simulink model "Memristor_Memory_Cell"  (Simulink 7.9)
settings: Solver=ode113  StartTime=0.0  StopTime=10.0  RelTol=3e-14
undefined symbols (not defined in the file or in its folder): sigbuilder_block
libraries: fl_lib x11, nesl_utility x5, Memristor_lib x1, elec_lib x1

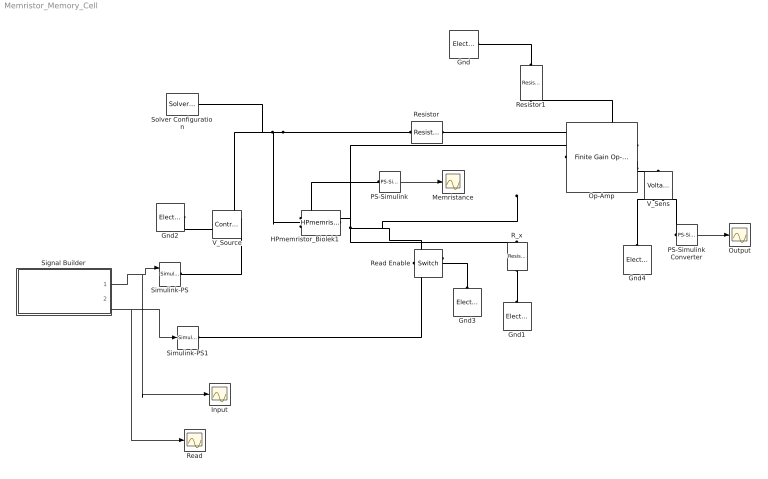
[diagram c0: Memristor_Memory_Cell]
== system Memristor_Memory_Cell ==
  Gnd{,1..4} (5 alike) : fl_lib/Electrical/Electrical Elements/Electrical Reference  i_Log=off  LocalVarNames=|i  LocalVarDescs=|i  LocalVarLogging=0
  HPmemristor_Biolek1 : Memristor_lib/HPmemristor_Biolek  R_off=500 Ohm  R_on=2 Ohm  pp=10 m  u_v=2.5e-15 m^2/s/V  D=1e-8 m  w0=10e-9 m  i_Log=off  v_Log=off  w_Log=off  F_Log=off  M_Log=off  LocalVarNames=|i|v|w|F|M  LocalVarDescs=|i|v|w|F|M  LocalVarLogging=[0 0 0 0 0]
  Input : Scope
  Memristance : Scope
  Op-Amp : elec_lib/Integrated Circuits/Finite Gain Op-Amp  A=10000  Rin=1e+6 Ohm  Rout=100 Ohm  Vmin=-.001 V  Vmax=5 V  LocalVarLogging=[]
  Output : Scope
  PS-Simulink : nesl_utility/PS-Simulink Converter  PhysicalDomain=network_engine_domain  LeftPortType=input  RightPortType=output  SubClassName=ps_output  Unit=1  AffineConversion=off
  PS-Simulink Converter : nesl_utility/PS-Simulink Converter  PhysicalDomain=network_engine_domain  LeftPortType=input  RightPortType=output  SubClassName=ps_output  Unit=1  AffineConversion=off
  R_x : fl_lib/Electrical/Electrical Elements/Resistor  R=52 Ohm  i_Log=off  v_Log=off  LocalVarNames=|i|v  LocalVarDescs=|i|v  LocalVarLogging=[0 0]
  Read : Scope
  Read Enable : fl_lib/Electrical/Electrical Elements/Switch  R_closed=.1e9 Ohm  G_open=100 1/Ohm  Threshold=1  i_Log=off  v_Log=off  LocalVarNames=|i|v  LocalVarDescs=|i|v  LocalVarLogging=[0 0]
  Resistor : fl_lib/Electrical/Electrical Elements/Resistor  R=2 Ohm  i_Log=off  v_Log=off  LocalVarNames=|i|v  LocalVarDescs=|i|v  LocalVarLogging=[0 0]
  Resistor1 : fl_lib/Electrical/Electrical Elements/Resistor  R=2 Ohm  i_Log=off  v_Log=off  LocalVarNames=|i|v  LocalVarDescs=|i|v  LocalVarLogging=[0 0]
  Signal Builder : Subsystem  Tag=STV Subsys  LoadFcn=sigbuilder_block('load');  StartFcn=sigbuilder_block('start');  StopFcn=sigbuilder_block('stop');  ClipboardFcn=sigbuilder_block('clipboard');
  Simulink-PS : nesl_utility/Simulink-PS Converter  PhysicalDomain=network_engine_domain  LeftPortType=input  RightPortType=output  SubClassName=ps_input  Unit=1  AffineConversion=off  InputFilterTimeConstant=.001  UdotUserProvided=2  SimscapeFilterOrder=1  InputFiltering=derivs
  Simulink-PS1 : nesl_utility/Simulink-PS Converter  PhysicalDomain=network_engine_domain  LeftPortType=input  RightPortType=output  SubClassName=ps_input  Unit=1  AffineConversion=off  InputFilterTimeConstant=.001  UdotUserProvided=0  SimscapeFilterOrder=1  InputFiltering=off
  Solver Configuration : nesl_utility/Solver Configuration  PhysicalDomain=network_engine_domain  LeftPortType=input  RightPortType=generic  SubClassName=solver  UseCustomDae=off  DoDC=off  ResidualTolerance=1e-9  UseLocalSolver=off  LocalSolverChoice=NE_BACKWARD_EULER_ADVANCER  LocalSolverSampleTime=.001  DoFixedCost=off  MaxNonlinIter=3  MaxModeIter=2  LinearAlgebra=Sparse  Accelerate=off  Profile=off  UseLocalSampling=off  DelaysMemoryBudget=1024
  V_Sens : fl_lib/Electrical/Electrical Sensors/Voltage Sensor  i1_Log=off  v1_Log=off  LocalVarNames=|i1|v1  LocalVarDescs=|i1|v1  LocalVarLogging=[0 0]
  V_Source : fl_lib/Electrical/Electrical Sources/Controlled Voltage Source  i_Log=off  v_Log=off  LocalVarNames=|i|v  LocalVarDescs=|i|v  LocalVarLogging=[0 0]
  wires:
  PS-Simulink Converter/1 -> Output/1
  PS-Simulink/1 -> Memristance/1
  Signal Builder/2(Read Enable) -> Simulink-PS1/1, Read/1
  Signal Builder/1(Signal Pulses) -> Simulink-PS/1, Input/1
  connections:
  R_x/LConn1 -- Op-Amp/LConn1 -- HPmemristor_Biolek1/RConn1 -- Read Enable/RConn2
  Op-Amp/LConn2 -- Resistor1/RConn1 -- Resistor/RConn1
  Resistor1/LConn1 -- Gnd/LConn1
  Gnd4/LConn1 -- V_Sens/RConn2
  PS-Simulink Converter/LConn1 -- V_Sens/RConn1
  V_Source/RConn1 -- Simulink-PS/RConn1
  Gnd2/LConn1 -- V_Source/RConn2
  Gnd1/LConn1 -- R_x/RConn1
  HPmemristor_Biolek1/RConn2 -- PS-Simulink/LConn1
  Resistor/LConn1 -- V_Source/LConn1 -- HPmemristor_Biolek1/LConn1 -- Solver Configuration/RConn1
  Read Enable/RConn1 -- Simulink-PS1/RConn1
  Op-Amp/RConn1 -- V_Sens/LConn1
  Gnd3/LConn1 -- Read Enable/LConn1

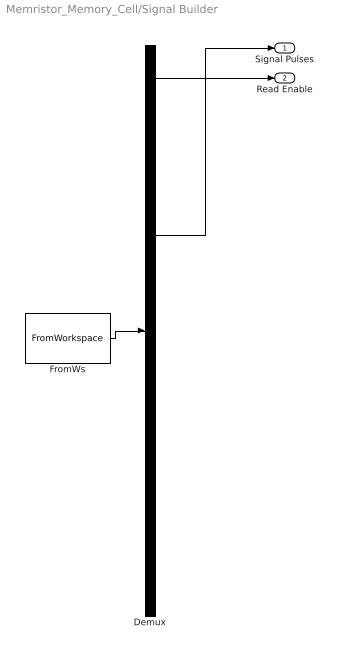
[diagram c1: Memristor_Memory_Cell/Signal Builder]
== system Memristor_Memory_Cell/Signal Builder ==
  Demux : Demux  Tag=STV Demux  Outputs=2
  FromWs : FromWorkspace  Tag=STV FromWs  VariableName=tuvar  SampleTime=0  SigBuilderData=DataTag0  VnvData=DataTag1
  Signal Pulses : Outport  Tag=STV Outport
  Read Enable : Outport  Tag=STV Outport  Port=2
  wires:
  Demux/1 -> Signal Pulses/1
  FromWs/1 -> Demux/1
  Demux/2 -> Read Enable/1
